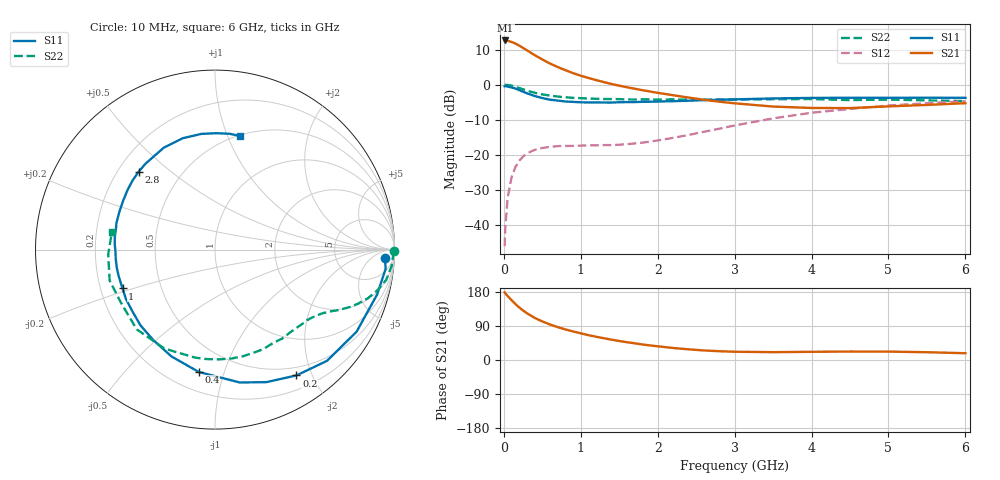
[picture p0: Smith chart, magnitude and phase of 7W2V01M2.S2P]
! Infineon Technologies  Discrete & RF Semiconductors
! BFS17W
! Si NPN RF Bipolar Junction Transistor in SOT323
! VCE = 2 V  IC = 1.2 mA
! Common Emitter S-Parameters:  August  1999
# GHz  S  MA  R  50
!  f  S11  S21  S12  S22
! GHz  MAG  ANG  MAG  ANG  MAG  ANG  MAG  ANG
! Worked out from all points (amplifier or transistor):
!   36 points, 10 MHz to 6 GHz, reference 50 ohm
!   highest |S21| = 12.6 dB at 20 MHz (marker M1)
!   |S21| within 3 dB of that: start of sweep to 313.9 MHz
!   unconditionally stable (mu >= 1): 948.7 MHz to end of sweep
!   at 250 MHz: K = 0.29, MSG = 15.5 dB, |S12| = -20.6 dB
!   at 1.4 GHz: K = 1.33, MAG = 5.3 dB, |S12| = -17.3 dB
!   at 6 GHz: K = 1.11, MAG = -2.3 dB, |S12| = -4.8 dB
!   S11 on the Smith chart (normalised r, x): 10 MHz: 20, -19; 200 MHz: 0.38, -1.77; 400 MHz: 0.32, -0.83; 1 GHz: 0.29, -0.18; 2.8 GHz: 0.28, +0.39; 6 GHz: 0.51, +1.11
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0.01  0.9479 -2.9  4.269 178.5  0.0049 84.8  0.999 -0.6
0.02  0.9567 -6.4  4.285 175.6  0.0093 83.2  0.9929 -2.0
0.05  0.9372 -15.5  4.233 168.6  0.0243 81.5  0.9889 -5.2
0.1  0.9119 -30.1  4.078 158.1  0.0468 72.8  0.9685 -10.1
0.15  0.8795 -44.8  3.876 147.7  0.0662 64.6  0.9315 -14.2
0.2  0.8351 -57.1  3.625 138.7  0.0817 58.6  0.8944 -17.6
0.25  0.792 -68.8  3.35 130.6  0.0936 52.5  0.8558 -20.4
0.3  0.7533 -79.4  3.101 123.5  0.1041 48.2  0.8236 -22.7
0.4  0.6879 -97.5  2.648 111.3  0.1167 41.0  0.766 -26.1
0.5  0.6428 -112.2  2.293 101.8  0.1243 36.5  0.7257 -28.4
0.6  0.61 -124.4  2.003 93.6  0.1288 33.6  0.6966 -30.6
0.8  0.5743 -143.4  1.611 80.7  0.1328 30.6  0.6596 -35.1
1  0.5588 -157.2  1.342 70.4  0.1344 30.8  0.6413 -39.5
1.1  0.5566 -164.1  1.246 65.5  0.1356 31.5  0.6335 -42.3
1.6  0.5632 171.9  0.917 46.9  0.1407 39.5  0.615 -56.3
2.2  0.5801 151.7  0.706 31.7  0.1734 52.3  0.6144 -74.8
2.8  0.6078 134.3  0.571 23.2  0.2347 58.1  0.6118 -94.4
3.5  0.6354 116.7  0.486 20.7  0.3296 56.0  0.6192 -117.1
4  0.646 106.1  0.464 21.6  0.3965 50.6  0.6225 -134.5
4.5  0.6492 96.6  0.462 22.4  0.4488 44.3  0.6018 -150.2
5.5  0.6506 82.8  0.513 20.5  0.5426 32.0  0.5956 -177.5
6  0.6482 77.7  0.543 17.9  0.5786 26.2  0.5827 170.4
